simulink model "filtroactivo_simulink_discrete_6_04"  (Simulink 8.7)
settings: Solver=ode45  StartTime=0.0  StopTime=stopTime  RelTol=1e-3
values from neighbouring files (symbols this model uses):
  C_LPF = 90e-6;5e-6;1e-6    [filtroactivo_simulink_discrete_6_default_values.m]    (also in filtroactivo_simulink_opt16_default_values.m; filtroactivo_LPF_C.m = 5.7e-06; filtroactivo_LPF_C_1.m = C; filtroactivo_LPF_C_2.m = 1.67e-05)
  close_net_switch_time = 1    [filtroactivo_simulink_discrete_6_default_values.m]
  control_current_start_time = close_net_switch_time    (= 1)    [filtroactivo_simulink_discrete_6_default_values.m]
  Iload_dephase = 0*pi/180 * [1 0 0 0 0 0 0]    [filtroactivo_simulink_discrete_6_default_values.m]    (also in filtroactivo_simulink_opt16_default_values.m)
  Iload_freq = 50*[1 5 7 11 13 17 19]    [filtroactivo_simulink_discrete_6_default_values.m]    (also in filtroactivo_simulink_opt16_default_values.m)
  Iload_peak = 16*sqrt(2)/100*[100 10 10 10 10 0 0]    [filtroactivo_simulink_discrete_6_default_values.m]    (also in filtroactivo_simulink_opt16_default_values.m)
  Iload_sampletime = 1e-6    (= 1e-06)    [filtroactivo_simulink_discrete_6_default_values.m]    (also in filtroactivo_simulink_opt16_default_values.m)
  Iload_simetric = [-1 1 -1 1 -1 1 -1]    [filtroactivo_simulink_discrete_6_default_values.m]    (also in filtroactivo_simulink_opt16_default_values.m)
  k_I_dqPLL = 0.05/pi    (= 0.0159154943092)    [filtroactivo_simulink_discrete_6_default_values.m]
  k_I_DVcc = 1e-3;1e-1    [filtroactivo_simulink_discrete_6_default_values.m]
  k_P_dqPLL = 0.05/pi    (= 0.0159154943092)    [filtroactivo_simulink_discrete_6_default_values.m]
  k_P_DVcc = 1e-4;2.5e-4;1e-2    [filtroactivo_simulink_discrete_6_default_values.m]
  L_grid = 15e-6    (= 1.5e-05)    [filtroactivo_simulink_discrete_6_default_values.m]    (also in filtroactivo_simulink_opt16_default_values.m; filtroactivo_LPF_C_2.m)
  L_LPF = L    (= 0.004)    [filtroactivo_LPF_C.m]    (also in filtroactivo_LPF_C_1.m = L; filtroactivo_LPF_L.m = 0.001)
  loopPeriod = period_control_current    [filtroactivo_simulink_discrete_6_default_values.m]
  period_control_plant = 0.5e-6    (= 5e-07)    [filtroactivo_simulink_discrete_6_default_values.m]
  period_control_switch = 2e-6    (= 2e-06)    [filtroactivo_simulink_discrete_6_default_values.m]
  R_C_LPF = .1;.5    [filtroactivo_simulink_discrete_6_default_values.m]    (also in filtroactivo_simulink_opt16_default_values.m; filtroactivo_LPF_C.m = 0.5; filtroactivo_LPF_C_2.m = 0.5)
  R_grid = 20e-3    (= 0.02)    [filtroactivo_simulink_discrete_6_default_values.m]    (also in filtroactivo_simulink_opt16_default_values.m; filtroactivo_LPF_C_2.m)
  R_L_LPF = .65;.125    [filtroactivo_simulink_discrete_6_default_values.m]    (also in filtroactivo_simulink_opt16_default_values.m; filtroactivo_LPF_C.m = 0.5)
  R_neutro_inverter_C_LPF = 1e-2;1;50;1e-2    [filtroactivo_simulink_discrete_6_default_values.m]    (also in filtroactivo_simulink_opt16_default_values.m)
  Vcc_desired = 900    [filtroactivo_simulink_discrete_6_default_values.m]    (also in filtroactivo_simulink_opt16_default_values.m)
  Vnet_dephase = 0*pi/180    (= 0)    [filtroactivo_simulink_discrete_6_default_values.m]    (also in filtroactivo_simulink_opt16_default_values.m)
  Vnet_freq = 50    [filtroactivo_simulink_discrete_6_default_values.m]    (also in filtroactivo_simulink_opt16_default_values.m)
  Vnet_peak = 566    [filtroactivo_simulink_discrete_6_default_values.m]    (also in filtroactivo_simulink_opt16_default_values.m)
undefined symbols (not defined in the file or in its folder): period_control_current
libraries: powerlib x50

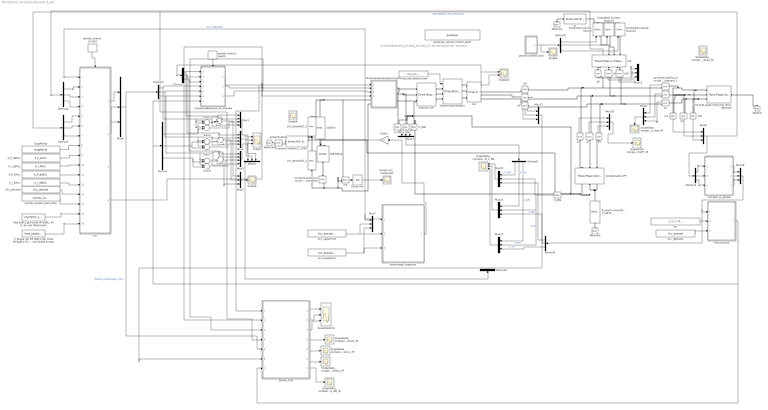
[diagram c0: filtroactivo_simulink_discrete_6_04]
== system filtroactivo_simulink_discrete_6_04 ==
  note: tic,sim('filtroactivo_simulink_discrete_2');,toc load gong.mat; sound(y);
  50Ohm : powerlib/Elements/Series RLC Branch  LConnTagsString=__new0  RConnTagsString=__new0  BranchType=R  Resistance=50  Inductance=1e-3  SetiL0=off  InitialCurrent=0  Capacitance=1e-6  Setx0=off  InitialVoltage=0  Measurements=None
  Condensator LPF : powerlib/Elements/Three-Phase Series RLC Branch  LConnTagsString=A|B|C  RConnTagsString=A|B|C  BranchType=RC  Resistance=R_C_LPF  Inductance=1e-3  Capacitance=C_LPF  Measurements=None
  Controlled Current Source : powerlib/Electrical Sources/Controlled Current Source  Initialize=off  Source_Type=AC  Amplitude=0  Phase=0  Frequency=0  Measurements=None
  Controlled Current Source1 : powerlib/Electrical Sources/Controlled Current Source  Initialize=off  Source_Type=AC  Amplitude=0  Phase=0  Frequency=0  Measurements=None
  Controlled Current Source2 : powerlib/Electrical Sources/Controlled Current Source  Initialize=off  Source_Type=AC  Amplitude=0  Phase=0  Frequency=0  Measurements=None
  Delay Vdc : UnitDelay  InitialCondition=Vcc_desired  SampleTime=-1
  Demux{,1..9} (10 alike) : Demux  Outputs=3
  Gain1 : Gain
  Grid Vnet_peak Vnet_freq Vnet_dephase : powerlib/Electrical Sources/Three-Phase Source  InternalConnection=Yn  VoltagePhases=off  Voltage=Vnet_peak/sqrt(2)  PhaseAngle=Vnet_dephase/pi*180  Voltage_phases=[25e3 25e3 25e3]/sqrt(3)  PhaseAngles_phases=[0 -120 +120]  Frequency=Vnet_freq  NonIdealSource=on  SpecifyImpedance=off  Resistance=R_grid  Inductance=L_grid  ShortCircuitLevel=100e6  BaseVoltage=25e3  XRratio=7  BusType=swing  Pref=0  Qref=0  Prefabc=[10e3, 10e3, 10e3]  Qrefabc=[0, 0, 0]  Qmin=-inf  Qmax=inf
  HB_calculus : MATLAB Function  TreatAsAtomicUnit=on
  IGBT/Diode : powerlib/Power Electronics/IGBT//Diode  Ron=1e-3  Rs=1e5  Cs=inf  Measurements=off
  Inductor LPF : powerlib/Elements/Three-Phase Series RLC Branch  LConnTagsString=A|B|C  RConnTagsString=A|B|C  BranchType=RL  Resistance=R_L_LPF  Inductance=L_LPF  Capacitance=1e-6  Measurements=None
  MOVIE_FCN : MATLAB Function  TreatAsAtomicUnit=on
  Mux1 : Mux
  Mux{5..18} (14 alike) : Mux  Inputs=3
  Mux2 : Mux
  Mux3 : Mux
  Neutral : powerlib/Elements/Neutral  LConnTagsString=a  NodeNumber=1
  Neutral1 : powerlib/Elements/Neutral  LConnTagsString=a  NodeNumber=2
  Neutral2 : powerlib/Elements/Neutral  LConnTagsString=a  NodeNumber=2
  Neutral4 : powerlib/Elements/Neutral  LConnTagsString=a  NodeNumber=2
  R : powerlib/Elements/Series RLC Branch  LConnTagsString=__new0  RConnTagsString=__new0  BranchType=R  Resistance=1  Inductance=1e-3  SetiL0=off  InitialCurrent=0  Capacitance=1e-6  Setx0=off  InitialVoltage=0  Measurements=None
  R_neutro_inverter_C_LPF/2 : powerlib/Elements/Series RLC Branch  LConnTagsString=__new0  RConnTagsString=__new0  BranchType=R  Resistance=R_neutro_inverter_C_LPF/2  Inductance=1e-3  SetiL0=off  InitialCurrent=0  Capacitance=1e-6  Setx0=off  InitialVoltage=0  Measurements=None
  R_neutro_inverter_C_LPF/2 _ : powerlib/Elements/Series RLC Branch  LConnTagsString=__new0  RConnTagsString=__new0  BranchType=R  Resistance=R_neutro_inverter_C_LPF/2  Inductance=1e-3  SetiL0=off  InitialCurrent=0  Capacitance=1e-6  Setx0=off  InitialVoltage=0  Measurements=None
  Scope1 : Scope
  Scope10 : Scope  NumInputPorts=2
  Scope4 : Scope
  Scope6 : Scope
  Scope7 : Scope  NumInputPorts=3
  ScopeData_compensator_Subsystem__Scope_HB_3F : Scope
  ScopeData_compensator_Subsystem__Scope_ICLPF_3F : Scope
  ScopeData_compensator_Subsystem__Scope_Iinversor_3F : Scope
  ScopeData_compensator_Subsystem__Scope_Iinversorreference_3F : Scope
  ScopeData_compensator_Subsystem__Scope_Iload_3F : Scope
  ScopeData_compensator_Subsystem__Scope_Inet_3F : Scope
  ScopeData_compensator_Subsystem__Scope_V_UN_V_MN_V_RN : Scope  NumInputPorts=3
  ScopeData_compensator_Subsystem__Scope_Vnet_measured_3F : Scope
  ScopeSwitchs : Scope  NumInputPorts=3
  Scope_Vcc_measured : Scope
  Sum1 : Sum  Inputs=+-
  Sum2 : Sum  Inputs=-+|
  Sum3 : Sum
  Sum4 : Sum  Inputs=-+|
  Sum5 : Sum  Inputs=-+|
  Sum6 : Sum  Inputs=+-
  Sum7 : Sum
  Sum8 : Sum  Inputs=+-
  Sum9 : Sum
  Three-Phase Breaker : powerlib/Elements/Three-Phase Breaker  InitialState=open  SwitchA=on  SwitchB=on  SwitchC=on  SwitchTimes=[0.020]  External=on  BreakerResistance=0.001  SnubberResistance=1e6  SnubberCapacitance=inf  Measurements=None
  Three-phase two-level inverter : Subsystem
  V_MN : powerlib/Measurements/Voltage Measurement  PhasorSimulation=off  OutputType=Complex  PSBequivalent=0
  V_UN : powerlib/Measurements/Voltage Measurement  PhasorSimulation=off  OutputType=Complex  PSBequivalent=0
  V_VN : powerlib/Measurements/Voltage Measurement  PhasorSimulation=off  OutputType=Complex  PSBequivalent=0
  V_WN : powerlib/Measurements/Voltage Measurement  PhasorSimulation=off  OutputType=Complex  PSBequivalent=0
  "V_phase-net Vd dqPLL got noise till dqPLL fix it, we use Vpeak known" : Constant  Value=Vnet_peak/sqrt(3)
  Vcc_desired : Constant  Value=Vcc_desired
  Vcc_desired/2_1 : powerlib/Elements/Series RLC Branch  LConnTagsString=__new0  RConnTagsString=__new0  BranchType=C  Resistance=0  Inductance=0  SetiL0=off  InitialCurrent=0  Capacitance=1e-2  Setx0=on  InitialVoltage=Vcc_desired/2  Measurements=None
  Vcc_desired/2_2 : powerlib/Elements/Series RLC Branch  LConnTagsString=__new0  RConnTagsString=__new0  BranchType=C  Resistance=0  Inductance=0  SetiL0=off  InitialCurrent=0  Capacitance=1e-2  Setx0=on  InitialVoltage=Vcc_desired/2  Measurements=None
  Vcc_desired1 : Constant  Value=Vcc_desired
  Vcc_lowerlimit : Constant  Value=Vcc_desired * 101 / 100
  Vcc_upperlimit : Constant  Value=Vcc_desired * 105 / 100
  a{,1..10} (11 alike) : powerlib/Measurements/Current Measurement  PhasorSimulation=off  OutputType=Complex  PSBequivalent=0
  amperimeter4 : powerlib/Measurements/Current Measurement  PhasorSimulation=off  OutputType=Complex  PSBequivalent=0
  close_net_switch_time : Constant  Value=close_net_switch_time
  complex_to_phase : MATLAB Function  TreatAsAtomicUnit=on
  control_current_start_time : Constant  Value=control_current_start_time
  "corriente positiva si va del + al - del block Current Measurement " : powerlib/Measurements/Current Measurement  PhasorSimulation=off  OutputType=Complex  PSBequivalent=0
  corriente positiva si va del + al - del block Current Measurement 1 : powerlib/Measurements/Current Measurement  PhasorSimulation=off  OutputType=Complex  PSBequivalent=0
  fcn : Subsystem
  "freq dqPLL got noise till dqPLL fix it, we use freq known" : Constant  Value=2*pi*50*C_LPF
  kH : Constant  Value=1 / ( 2 * 0.005 * 25e3 *Vcc_desired )
  k_I_DVcc : Constant  Value=k_I_dqPLL
  k_I_dqPLL : Constant  Value=k_I_DVcc
  k_P_DVcc : Constant  Value=k_P_dqPLL
  k_P_dqPLL : Constant  Value=k_P_DVcc
  loopPeriod : Constant  Value=loopPeriod
  m{1,3,5,8} (4 alike) : powerlib/Measurements/Voltage Measurement  PhasorSimulation=off  OutputType=Complex  PSBequivalent=0
  m2 : powerlib/Measurements/Three-Phase V-I Measurement  VoltageMeasurement=phase-to-phase  SetLabelV=off  LabelV=Vabc  Vpu=off  VpuLL=off  CurrentMeasurement=yes  SetLabelI=off  LabelI=Iabc  Ipu=off  Pbase=100e6  Vbase=500e3  OutputType=Complex  PhasorSimulation=off  PSBequivalent=0
  m6 : powerlib/Measurements/Three-Phase V-I Measurement  VoltageMeasurement=phase-to-phase  SetLabelV=off  LabelV=Vabc  Vpu=off  VpuLL=off  CurrentMeasurement=yes  SetLabelI=off  LabelI=Iabc  Ipu=off  Pbase=100e6  Vbase=500e3  OutputType=Complex  PhasorSimulation=off  PSBequivalent=0
  measured&desired_to_SuSvSw : Subsystem
  overcharge_capacitor : MATLAB Function  TreatAsAtomicUnit=on
  period_control_current : DiscretePulseGenerator  PulseType=Time based  Period=period_control_current  PulseWidth=50
  period_control_switch : DiscretePulseGenerator  PulseType=Time based  Period=period_control_switch  PulseWidth=50
  phase currents load : Subsystem
  powergui_period_control_plant : powerlib/powergui  Priority=1  SimulationMode=Discrete  SolverType=Tustin  SampleTime=period_control_plant  frequency=60  SPID=off  DisableSnubberDevices=off  DisableRonSwitches=off  DisableVfSwitches=off  SwTol=0  DisplayEquations=off  Interpol=off  ExternalGateDelay=off  methode=off  Ts=10  FunctionMessages=off  echomessages=off  HookPort=off  EnableUseOfTLC=off  x0status=blocks  frequencyindice=0  Pbase=100e6  ErrMax=1e-4  Iterations=50  UnitsV=kV  UnitsW=MW  buscounter=0  RestoreLinks=warning  ResistiveCurrentMeasurement=off  Frange=[0:2:500]  Ylog=off  Xlog=on  ShowGrid=off  save=off  variable=ZData  structure=ScopeData_compensator_Subsystem__Scope11  ZoomFFT=off  StartTime=4.72  cycles=14  DisplayStyle=3  fundamental=50  FreqAxis=on  MaxFrequency=40*50  frequencyindicesteady=1  RmsSteady=1  display=off
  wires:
  period_control_switch/1 -> measured&desired_to_SuSvSw/Trigger
  Demux2/1 -> measured&desired_to_SuSvSw/4(Iu*), Sum2/2, Mux1/2, Sum1/1, Sum3/1
  Demux2/2 -> measured&desired_to_SuSvSw/5(Iv*), Sum7/1, Sum6/1, Mux2/2, Sum4/2
  Demux2/3 -> measured&desired_to_SuSvSw/6(Iw*), Sum9/1, Sum8/1, Mux3/2, Sum5/2
  Mux1/1 -> Mux16/1, Scope7/1
  Sum1/1 -> Mux1/4
  Sum3/1 -> Mux1/3
  Mux2/1 -> Scope7/2, Mux16/2
  Mux3/1 -> Mux16/3, Scope7/3
  Sum6/1 -> Mux2/3
  Sum8/1 -> Mux3/3
  Demux/1 -> Sum1/2, Sum3/2
  Demux/2 -> Sum6/2, Sum7/2
  Demux/3 -> Sum9/2, Sum8/2
  m3/1 -> Delay Vdc/1
  HB_calculus/1(HB) -> MOVIE_FCN/7(g), Demux/1, measured&desired_to_SuSvSw/7(H)
  m2/1 -> Scope10/2
  Mux9/1 -> MOVIE_FCN/4(d), Demux7/1, Demux3/1  "Vphasephase_net_measured"
  Demux1/2 -> Sum4/1, Mux2/1, measured&desired_to_SuSvSw/2(Iv)
  Demux1/3 -> measured&desired_to_SuSvSw/3(Iw), Sum5/1, Mux3/1
  Demux1/1 -> Sum2/1, Mux1/1, measured&desired_to_SuSvSw/1(Iu)
  Demux5/1 -> Controlled Current Source/1
  Demux5/2 -> Controlled Current Source1/1
  Demux5/3 -> Controlled Current Source2/1
  phase currents load/1(Out1) -> Scope1/1, Demux5/1
  Mux5/1 -> Scope6/1
  Sum2/1 -> Mux5/1
  Sum4/1 -> Mux5/2
  Sum5/1 -> Mux5/3
  Sum7/1 -> Mux2/4
  Sum9/1 -> Mux3/4
  m2/2 -> Scope10/1, Demux1/1
  Mux6/1 -> MOVIE_FCN/5(e), Demux2/1  "Iphase_compensator_reference"
  amperimeter4/1 -> ?
  Delay Vdc/1 -> fcn/1(Vcc_measured), Scope_Vcc_measured/1, overcharge_capacitor/1(Vcc_measured), Mux7/1  "Vcc_measured"
  period_control_current/1 -> fcn/Trigger
  fcn/2(Iv_ref) -> Mux6/2
  fcn/3(Iw_ref) -> Mux6/3
  fcn/1(Iu_ref) -> Mux6/1
  m6/2 -> Demux4/1
  Demux4/1 -> fcn/2(Ia_load)
  close_net_switch_time/1 -> Three-Phase Breaker/1
  fcn/4(activate_poles) -> Three-phase two-level inverter/4(activate_poles)
  Vcc_upperlimit/1 -> overcharge_capacitor/2(Vcc_upperlimit), Mux7/2
  Vcc_lowerlimit/1 -> overcharge_capacitor/3(Vcc_lowerlimit), Mux7/3
  overcharge_capacitor/1(pSfrenado) -> Gain1/1
  Gain1/1 -> IGBT/Diode/1
  Mux7/1 -> ?
  "corriente positiva si va del + al - del block Current Measurement "/1 -> ?
  Mux8/1 -> ScopeData_compensator_Subsystem__Scope_Inet_3F/1
  corriente positiva si va del + al - del block Current Measurement 1/1 -> Mux8/1
  a/1 -> Mux8/2
  a1/1 -> Mux8/3
  m1/1 -> Mux9/1
  m5/1 -> Mux9/2
  m8/1 -> Mux9/3
  Mux10/1 -> ScopeData_compensator_Subsystem__Scope_ICLPF_3F/1
  a2/1 -> Mux10/1
  a3/1 -> Mux10/2
  a4/1 -> Mux10/3
  Mux11/1 -> MOVIE_FCN/6(f)
  a5/1 -> Mux11/1
  a6/1 -> Mux11/2
  a7/1 -> Mux11/3
  Mux12/1 -> ?
  a10/1 -> Mux12/3
  a9/1 -> Mux12/2
  a8/1 -> Mux12/1
  control_current_start_time/1 -> fcn/14(control_current_start_time)
  loopPeriod/1 -> fcn/8(loopPeriod)
  k_P_DVcc/1 -> fcn/11(k_P_dqPLL)
  k_I_DVcc/1 -> fcn/12(k_I_dqPLL)
  k_I_dqPLL/1 -> fcn/10(k_I_DVcc)
  k_P_dqPLL/1 -> fcn/9(k_P_DVcc)
  "freq dqPLL got noise till dqPLL fix it, we use freq known"/1 -> fcn/15(X_C_LPF)
  "V_phase-net Vd dqPLL got noise till dqPLL fix it, we use Vpeak known"/1 -> fcn/16(Vpeak_arbitrary)
  Vcc_desired/1 -> fcn/13(Vcc_desired)
  Demux4/2 -> fcn/3(Ib_load)
  Demux4/3 -> fcn/4(Ic_load)
  Demux7/1 -> fcn/5(Va)
  Demux7/2 -> fcn/6(Vb)
  Demux7/3 -> fcn/7(Vc)
  Mux13/1 -> ScopeData_compensator_Subsystem__Scope_V_UN_V_MN_V_RN/1
  Demux3/2 -> complex_to_phase/2(Vst)
  Demux3/1 -> complex_to_phase/1(Vrs)
  Demux3/3 -> complex_to_phase/3(Vtr)
  measured&desired_to_SuSvSw/3(Sw) -> MOVIE_FCN/3(c), Three-phase two-level inverter/3(Sc)
  measured&desired_to_SuSvSw/2(Sv) -> MOVIE_FCN/2(b), Three-phase two-level inverter/2(Sb)
  measured&desired_to_SuSvSw/1(Su) -> MOVIE_FCN/1(a), Three-phase two-level inverter/1(Sa)
  Mux14/1 -> ScopeData_compensator_Subsystem__Scope_V_UN_V_MN_V_RN/2
  Mux16/1 -> Demux6/1
  V_VN/1 -> Mux17/2
  V_WN/1 -> Mux17/3
  V_UN/1 -> Mux17/1
  V_MN/1 -> Mux15/2, Mux14/2, Mux13/2  "V_MN"
  Mux17/1 -> Demux8/1
  Demux8/1 -> Mux13/1  "V_UN"
  Demux8/2 -> Mux14/1  "V_VN"
  Demux8/3 -> Mux15/1  "V_WN"
  complex_to_phase/2(Vs) -> Mux18/2
  complex_to_phase/1(Vr) -> Mux18/1
  complex_to_phase/3(Vt) -> Mux18/3
  Mux18/1 -> Demux9/1, HB_calculus/1(Vfaseneutro)
  Demux9/1 -> Mux13/3  "V_RN"
  Demux9/2 -> Mux14/3  "V_SN"
  Demux9/3 -> Mux15/3  "V_TN"
  Demux6/1 -> ?  "I_U"
  Demux6/2 -> ?  "I_V"
  Demux6/3 -> ?  "I_W"
  Mux15/1 -> ScopeData_compensator_Subsystem__Scope_V_UN_V_MN_V_RN/3
  kH/1 -> HB_calculus/2(Kh)
  Vcc_desired1/1 -> HB_calculus/3(Vcc_desired)
  MOVIE_FCN/1(a1) -> ScopeSwitchs/1
  MOVIE_FCN/2(b1) -> ScopeSwitchs/2
  MOVIE_FCN/3(c1) -> ScopeSwitchs/3
  MOVIE_FCN/4(d1) -> ScopeData_compensator_Subsystem__Scope_Vnet_measured_3F/1
  MOVIE_FCN/5(e1) -> ScopeData_compensator_Subsystem__Scope_Iinversorreference_3F/1
  MOVIE_FCN/6(f1) -> ScopeData_compensator_Subsystem__Scope_Iinversor_3F/1
  MOVIE_FCN/7(g1) -> ScopeData_compensator_Subsystem__Scope_HB_3F/1
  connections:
  Vcc_desired/2_2/RConn1 -- "corriente positiva si va del + al - del block Current Measurement "/RConn1 -- Three-phase two-level inverter/LConn2 -- m3/LConn2
  Three-phase two-level inverter/LConn1 -- 50Ohm/RConn1 -- Vcc_desired/2_1/LConn1 -- m3/LConn1
  corriente positiva si va del + al - del block Current Measurement 1/RConn1 -- a8/RConn1 -- a2/RConn1 -- a5/RConn1
  Controlled Current Source/RConn1 -- Controlled Current Source1/RConn1 -- Controlled Current Source2/RConn1 -- R/RConn1
  a/RConn1 -- a9/RConn1 -- a3/RConn1 -- a6/RConn1
  a1/RConn1 -- a4/RConn1 -- a7/RConn1 -- a10/RConn1
  Condensator LPF/RConn2 -- V_WN/LConn2 -- V_VN/LConn2 -- V_UN/LConn2 -- V_MN/LConn2 -- Condensator LPF/RConn1 -- Condensator LPF/RConn3 -- R_neutro_inverter_C_LPF/2 _/RConn1
  Vcc_desired/2_1/RConn1 -- Vcc_desired/2_2/LConn1 -- V_MN/LConn1 -- R_neutro_inverter_C_LPF/2/RConn1
  Three-phase two-level inverter/RConn1 -- V_UN/LConn1 -- Inductor LPF/LConn1
  Three-phase two-level inverter/RConn2 -- V_VN/LConn1 -- Inductor LPF/LConn2
  m6/RConn1 -- Controlled Current Source/LConn1
  Neutral1/LConn1 -- R/LConn1
  Grid Vnet_peak Vnet_freq Vnet_dephase/RConn2 -- m1/LConn2 -- a/LConn1 -- m5/LConn1
  Grid Vnet_peak Vnet_freq Vnet_dephase/LConn1 -- Neutral/LConn1
  Inductor LPF/RConn3 -- Three-Phase Breaker/LConn3
  Inductor LPF/RConn1 -- Three-Phase Breaker/LConn1
  Grid Vnet_peak Vnet_freq Vnet_dephase/RConn1 -- m8/LConn2 -- m1/LConn1 -- corriente positiva si va del + al - del block Current Measurement 1/LConn1
  m2/LConn1 -- Three-Phase Breaker/RConn1
  m6/RConn2 -- Controlled Current Source1/LConn1
  Inductor LPF/RConn2 -- Three-Phase Breaker/LConn2
  m2/LConn3 -- Three-Phase Breaker/RConn3
  m2/LConn2 -- Three-Phase Breaker/RConn2
  m6/RConn3 -- Controlled Current Source2/LConn1
  R_neutro_inverter_C_LPF/2 _/LConn1 -- Neutral2/LConn1
  Inductor LPF/LConn3 -- V_WN/LConn1 -- Three-phase two-level inverter/RConn3
  Grid Vnet_peak Vnet_freq Vnet_dephase/RConn3 -- m8/LConn1 -- m5/LConn2 -- a1/LConn1
  amperimeter4/LConn1 -- Neutral4/LConn1
  R_neutro_inverter_C_LPF/2/LConn1 -- amperimeter4/RConn1
  50Ohm/LConn1 -- IGBT/Diode/LConn1
  "corriente positiva si va del + al - del block Current Measurement "/LConn1 -- IGBT/Diode/RConn1
  a3/LConn1 -- Condensator LPF/LConn2
  Condensator LPF/LConn3 -- a4/LConn1
  a2/LConn1 -- Condensator LPF/LConn1
  a6/LConn1 -- m2/RConn2
  a5/LConn1 -- m2/RConn1
  a7/LConn1 -- m2/RConn3
  a8/LConn1 -- m6/LConn1
  a9/LConn1 -- m6/LConn2
  a10/LConn1 -- m6/LConn3

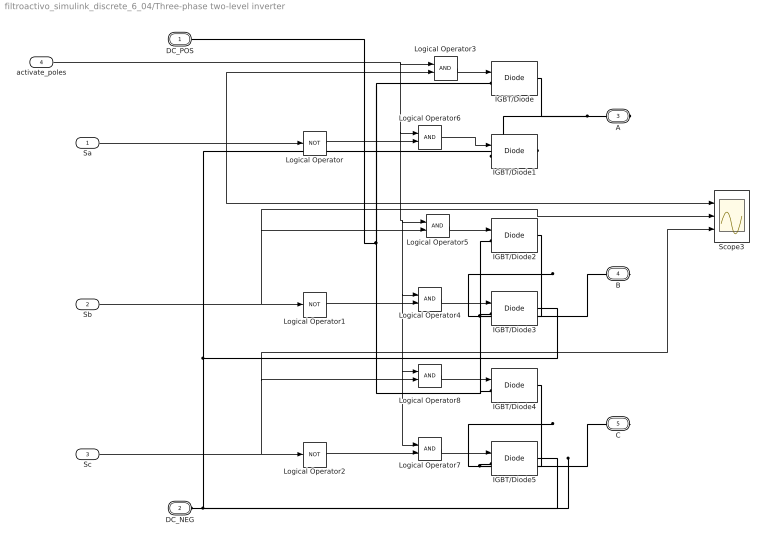
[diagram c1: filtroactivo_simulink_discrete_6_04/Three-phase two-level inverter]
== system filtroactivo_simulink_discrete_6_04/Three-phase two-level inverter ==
  Sa : Inport
  Sb : Inport  Port=2
  Sc : Inport  Port=3
  activate_poles : Inport  Port=4
  IGBT/Diode{,1..5} (6 alike) : powerlib/Power Electronics/IGBT//Diode  Ron=1e-3  Rs=1e5  Cs=inf  Measurements=off
  Logical Operator : Logic  Operator=NOT  AllPortsSameDT=off  OutDataTypeStr=boolean
  Logical Operator1 : Logic  Operator=NOT  AllPortsSameDT=off  OutDataTypeStr=boolean
  Logical Operator2 : Logic  Operator=NOT  AllPortsSameDT=off  OutDataTypeStr=boolean
  Logical Operator{3..8} (6 alike) : Logic  AllPortsSameDT=off  OutDataTypeStr=boolean
  Scope3 : Scope  NumInputPorts=3
  DC_POS : PMIOPort  Tag=PMCPort  Port=1  Side=Left
  DC_NEG : PMIOPort  Tag=PMCPort  Port=2  Side=Left
  A : PMIOPort  Tag=PMCPort  Port=3  Side=Right
  B : PMIOPort  Tag=PMCPort  Port=4  Side=Right
  C : PMIOPort  Tag=PMCPort  Port=5  Side=Right
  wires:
  Sc/1 -> Scope3/3, Logical Operator8/2, Logical Operator2/1
  Logical Operator2/1 -> Logical Operator7/2
  Sb/1 -> Scope3/2, Logical Operator5/2, Logical Operator1/1
  Sa/1 -> Scope3/1, Logical Operator3/2, Logical Operator/1
  activate_poles/1 -> Logical Operator6/1, Logical Operator7/1, Logical Operator8/1, Logical Operator4/1, Logical Operator5/1, Logical Operator3/1
  Logical Operator3/1 -> IGBT/Diode/1
  Logical Operator/1 -> Logical Operator6/2
  Logical Operator6/1 -> IGBT/Diode1/1
  Logical Operator1/1 -> Logical Operator4/2
  Logical Operator4/1 -> IGBT/Diode3/1
  Logical Operator5/1 -> IGBT/Diode2/1
  Logical Operator7/1 -> IGBT/Diode5/1
  Logical Operator8/1 -> IGBT/Diode4/1
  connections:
  IGBT/Diode5/LConn1 -- IGBT/Diode4/RConn1 -- C/RConn1
  IGBT/Diode3/LConn1 -- B/RConn1 -- IGBT/Diode2/RConn1
  IGBT/Diode4/LConn1 -- IGBT/Diode2/LConn1 -- DC_POS/RConn1 -- IGBT/Diode/LConn1
  A/RConn1 -- IGBT/Diode1/LConn1 -- IGBT/Diode/RConn1
  DC_NEG/RConn1 -- IGBT/Diode5/RConn1 -- IGBT/Diode3/RConn1 -- IGBT/Diode1/RConn1

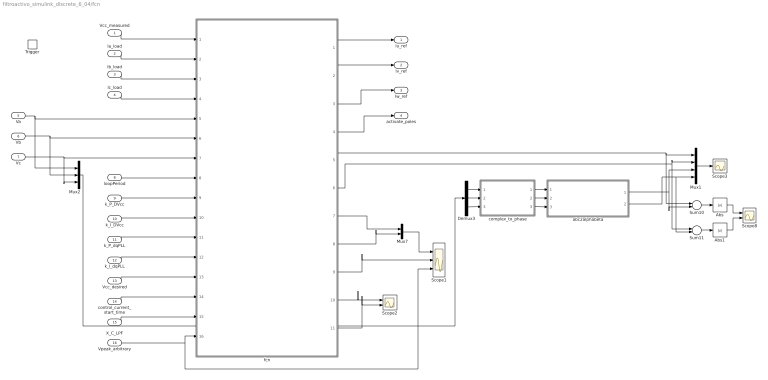
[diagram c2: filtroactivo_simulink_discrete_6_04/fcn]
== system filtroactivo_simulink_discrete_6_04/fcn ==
  Vcc_measured : Inport
  Ia_load : Inport  Port=2
  Ib_load : Inport  Port=3
  Ic_load : Inport  Port=4
  Va : Inport  Port=5
  Vb : Inport  Port=6
  Vc : Inport  Port=7
  loopPeriod : Inport  Port=8
  k_P_DVcc : Inport  Port=9
  k_I_DVcc : Inport  Port=10
  k_P_dqPLL : Inport  Port=11
  k_I_dqPLL : Inport  Port=12
  Vcc_desired : Inport  Port=13
  control_current_start_time : Inport  Port=14
  X_C_LPF : Inport  Port=15
  Vpeak_arbitrary : Inport  Port=16
  Trigger : TriggerPort  VariantControl=Variant
  Abs : Abs
  Abs1 : Abs
  Demux3 : Demux  Outputs=3
  Mux1 : Mux
  Mux2 : Mux  Inputs=3
  Mux7 : Mux  Inputs=2
  Scope1 : Scope  NumInputPorts=3
  Scope2 : Scope  NumInputPorts=2
  Scope3 : Scope
  Scope8 : Scope  NumInputPorts=2
  Sum10 : Sum  Inputs=+-
  Sum11 : Sum  Inputs=+-
  abc2alphabeta : MATLAB Function  TreatAsAtomicUnit=on
  complex_to_phase : MATLAB Function  TreatAsAtomicUnit=on
  fcn : MATLAB Function  TreatAsAtomicUnit=on
  Iu_ref : Outport
  Iv_ref : Outport  Port=2
  Iw_ref : Outport  Port=3
  activate_poles : Outport  Port=4
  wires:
  Vc/1 -> Mux2/3, fcn/7(Vc)
  Vb/1 -> Mux2/2, fcn/6(Vb)
  Ic_load/1 -> fcn/4(Ic_load)
  Va/1 -> Mux2/1, fcn/5(Va)
  Ib_load/1 -> fcn/3(Ib_load)
  Ia_load/1 -> fcn/2(Ia_load)
  Vcc_measured/1 -> fcn/1(Vcc_measured)
  loopPeriod/1 -> fcn/8(loopPeriod)
  k_P_DVcc/1 -> fcn/9(k_P_DVcc)
  k_I_DVcc/1 -> fcn/10(k_I_DVcc)
  Vpeak_arbitrary/1 -> fcn/16(Vpeak_arbitrary), Scope1/3
  fcn/2(Iv_ref) -> Iv_ref/1
  fcn/3(Iw_ref) -> Iw_ref/1
  fcn/4(activate_poles) -> activate_poles/1
  fcn/1(Iu_ref) -> Iu_ref/1
  Mux7/1 -> Scope1/1
  fcn/7(control_current_start_counter_output) -> Mux7/1
  fcn/8(control_current_start_counter_max_output) -> Mux7/2
  fcn/9(DVcc) -> Scope1/2
  fcn/10(DVcc_afterPI) -> Scope2/1
  fcn/11(PI_I_output) -> Scope2/2
  Demux3/1 -> complex_to_phase/1(Vrs)
  Demux3/2 -> complex_to_phase/2(Vst)
  Demux3/3 -> complex_to_phase/3(Vtr)
  complex_to_phase/1(Vr) -> abc2alphabeta/1(a)
  complex_to_phase/2(Vs) -> abc2alphabeta/2(b)
  complex_to_phase/3(Vt) -> abc2alphabeta/3(c)
  Mux1/1 -> Scope3/1
  fcn/6(V_beta) -> Mux1/2, Sum11/1
  fcn/5(V_alpha) -> Sum10/1, Mux1/1
  abc2alphabeta/1(alpha) -> Mux1/3, Sum10/2
  abc2alphabeta/2(beta) -> Sum11/2, Mux1/4
  Sum10/1 -> Abs/1
  Sum11/1 -> Abs1/1
  Abs1/1 -> Scope8/2
  Abs/1 -> Scope8/1
  Mux2/1 -> Demux3/1
  k_I_dqPLL/1 -> fcn/12(k_I_dqPLL)
  k_P_dqPLL/1 -> fcn/11(k_P_dqPLL)
  X_C_LPF/1 -> fcn/15(X_C_LPF)
  Vcc_desired/1 -> fcn/13(Vcc_desired)
  control_current_start_time/1 -> fcn/14(control_current_start_time)

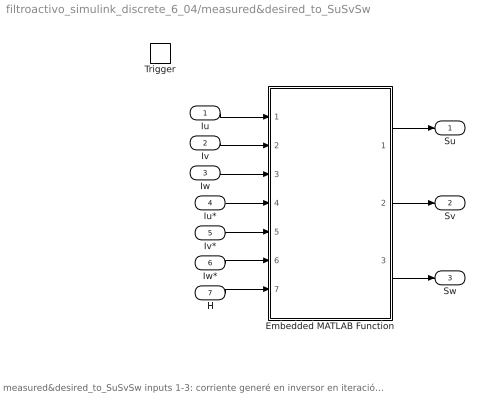
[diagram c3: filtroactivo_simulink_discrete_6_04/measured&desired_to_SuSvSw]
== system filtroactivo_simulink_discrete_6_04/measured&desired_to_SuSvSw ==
  note: measured&desired_to_SuSvSw inputs 1-3: corriente generé en inversor en iteración anterior inputs 4-6: corriente q deseo generar en inversor outputs: disparos Su,Sv,Sw q definen la corriente mas parecida a deseada que puedo generar
  Iu : Inport
  Iv : Inport  Port=2
  Iw : Inport  Port=3
  Iu* : Inport  Port=4
  Iv* : Inport  Port=5
  Iw* : Inport  Port=6
  H : Inport  Port=7
  Trigger : TriggerPort  VariantControl=Variant
  Embedded MATLAB Function : MATLAB Function  TreatAsAtomicUnit=on
  Su : Outport
  Sv : Outport  Port=2
  Sw : Outport  Port=3
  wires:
  Embedded MATLAB Function/3(Sw) -> Sw/1
  Embedded MATLAB Function/2(Sv) -> Sv/1
  Embedded MATLAB Function/1(Su) -> Su/1
  Iu/1 -> Embedded MATLAB Function/1(Iu)
  Iv/1 -> Embedded MATLAB Function/2(Iv)
  Iw/1 -> Embedded MATLAB Function/3(Iw)
  Iu*/1 -> Embedded MATLAB Function/4(Iu1)
  Iv*/1 -> Embedded MATLAB Function/5(Iv1)
  Iw*/1 -> Embedded MATLAB Function/6(Iw1)
  H/1 -> Embedded MATLAB Function/7(H)

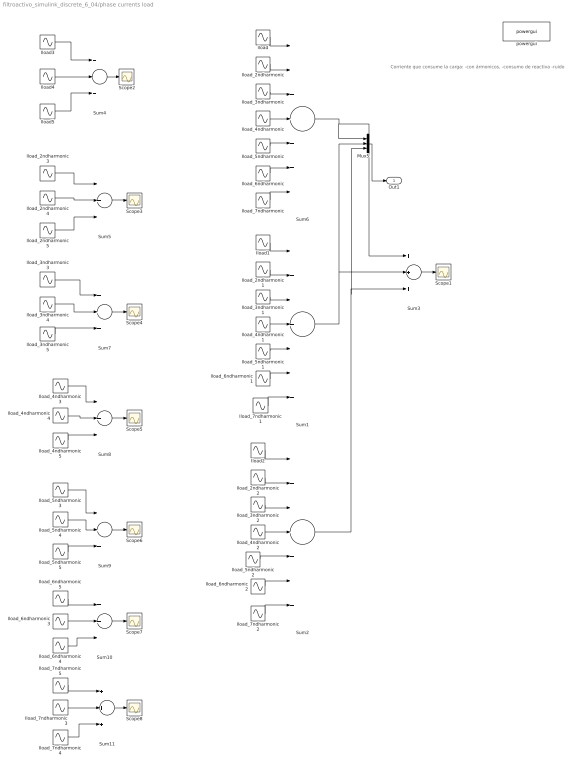
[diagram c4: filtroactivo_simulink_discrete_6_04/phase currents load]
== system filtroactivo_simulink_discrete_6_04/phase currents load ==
  note: Corriente que consume la carga: -con ármonicos, -consumo de reactiva -ruido
  Iload : Sin  Amplitude=Iload_peak(1)  Frequency=2*pi*Iload_freq(1)  Phase=Iload_dephase(1)  SampleTime=Iload_sampletime
  Iload1 : Sin  Amplitude=Iload_peak(1)  Frequency=2*pi*Iload_freq(1)  Phase=Iload_dephase(1) + 2*pi/3*Iload_simetric(1)  SampleTime=Iload_sampletime
  Iload2 : Sin  Amplitude=Iload_peak(1)  Frequency=2*pi*Iload_freq(1)  Phase=Iload_dephase(1) + 4*pi/3*Iload_simetric(1)  SampleTime=Iload_sampletime
  Iload3 : Sin  Amplitude=Iload_peak(1)  Frequency=2*pi*Iload_freq(1)  Phase=Iload_dephase(1)  SampleTime=Iload_sampletime
  Iload4 : Sin  Amplitude=Iload_peak(1)  Frequency=2*pi*Iload_freq(1)  Phase=Iload_dephase(1) + 2*pi/3*Iload_simetric(1)  SampleTime=Iload_sampletime
  Iload5 : Sin  Amplitude=Iload_peak(1)  Frequency=2*pi*Iload_freq(1)  Phase=Iload_dephase(1) + 4*pi/3*Iload_simetric(1)  SampleTime=Iload_sampletime
  Iload_2ndharmonic : Sin  Amplitude=Iload_peak(2)  Frequency=2*pi*Iload_freq(2)  Phase=Iload_dephase(2)  SampleTime=Iload_sampletime
  Iload_2ndharmonic1 : Sin  Amplitude=Iload_peak(2)  Frequency=2*pi*Iload_freq(2)  Phase=Iload_dephase(2) + 2*pi/3*Iload_simetric(2)  SampleTime=Iload_sampletime
  Iload_2ndharmonic2 : Sin  Amplitude=Iload_peak(2)  Frequency=2*pi*Iload_freq(2)  Phase=Iload_dephase(2) + 4*pi/3*Iload_simetric(2)  SampleTime=Iload_sampletime
  Iload_2ndharmonic3 : Sin  Amplitude=Iload_peak(2)  Frequency=2*pi*Iload_freq(2)  Phase=Iload_dephase(2)  SampleTime=Iload_sampletime
  Iload_2ndharmonic4 : Sin  Amplitude=Iload_peak(2)  Frequency=2*pi*Iload_freq(2)  Phase=Iload_dephase(2) + 2*pi/3*Iload_simetric(2)  SampleTime=Iload_sampletime
  Iload_2ndharmonic5 : Sin  Amplitude=Iload_peak(2)  Frequency=2*pi*Iload_freq(2)  Phase=Iload_dephase(2) + 4*pi/3*Iload_simetric(2)  SampleTime=Iload_sampletime
  Iload_3ndharmonic : Sin  Amplitude=Iload_peak(3)  Frequency=2*pi*Iload_freq(3)  Phase=Iload_dephase(3)  SampleTime=Iload_sampletime
  Iload_3ndharmonic1 : Sin  Amplitude=Iload_peak(3)  Frequency=2*pi*Iload_freq(3)  Phase=Iload_dephase(3) + 2*pi/3*Iload_simetric(3)  SampleTime=Iload_sampletime
  Iload_3ndharmonic2 : Sin  Amplitude=Iload_peak(3)  Frequency=2*pi*Iload_freq(3)  Phase=Iload_dephase(3) + 4*pi/3*Iload_simetric(3)  SampleTime=Iload_sampletime
  Iload_3ndharmonic3 : Sin  Amplitude=Iload_peak(3)  Frequency=2*pi*Iload_freq(3)  Phase=Iload_dephase(3)  SampleTime=Iload_sampletime
  Iload_3ndharmonic4 : Sin  Amplitude=Iload_peak(3)  Frequency=2*pi*Iload_freq(3)  Phase=Iload_dephase(3) + 2*pi/3*Iload_simetric(3)  SampleTime=Iload_sampletime
  Iload_3ndharmonic5 : Sin  Amplitude=Iload_peak(3)  Frequency=2*pi*Iload_freq(3)  Phase=Iload_dephase(3) + 4*pi/3*Iload_simetric(3)  SampleTime=Iload_sampletime
  Iload_4ndharmonic : Sin  Amplitude=Iload_peak(4)  Frequency=2*pi*Iload_freq(4)  Phase=Iload_dephase(4)  SampleTime=Iload_sampletime
  Iload_4ndharmonic1 : Sin  Amplitude=Iload_peak(4)  Frequency=2*pi*Iload_freq(4)  Phase=Iload_dephase(4) + 2*pi/3*Iload_simetric(4)  SampleTime=Iload_sampletime
  Iload_4ndharmonic2 : Sin  Amplitude=Iload_peak(4)  Frequency=2*pi*Iload_freq(4)  Phase=Iload_dephase(4) + 4*pi/3*Iload_simetric(4)  SampleTime=Iload_sampletime
  Iload_4ndharmonic3 : Sin  Amplitude=Iload_peak(4)  Frequency=2*pi*Iload_freq(4)  Phase=Iload_dephase(4)  SampleTime=Iload_sampletime
  Iload_4ndharmonic4 : Sin  Amplitude=Iload_peak(4)  Frequency=2*pi*Iload_freq(4)  Phase=Iload_dephase(4) + 2*pi/3*Iload_simetric(4)  SampleTime=Iload_sampletime
  Iload_4ndharmonic5 : Sin  Amplitude=Iload_peak(4)  Frequency=2*pi*Iload_freq(4)  Phase=Iload_dephase(4) + 4*pi/3*Iload_simetric(4)  SampleTime=Iload_sampletime
  Iload_5ndharmonic : Sin  Amplitude=Iload_peak(5)  Frequency=2*pi*Iload_freq(5)  Phase=Iload_dephase(5)  SampleTime=Iload_sampletime
  Iload_5ndharmonic1 : Sin  Amplitude=Iload_peak(5)  Frequency=2*pi*Iload_freq(5)  Phase=Iload_dephase(5) + 2*pi/3*Iload_simetric(5)  SampleTime=Iload_sampletime
  Iload_5ndharmonic2 : Sin  Amplitude=Iload_peak(5)  Frequency=2*pi*Iload_freq(5)  Phase=Iload_dephase(5) + 4*pi/3*Iload_simetric(5)  SampleTime=Iload_sampletime
  Iload_5ndharmonic3 : Sin  Amplitude=Iload_peak(5)  Frequency=2*pi*Iload_freq(5)  Phase=Iload_dephase(5)  SampleTime=Iload_sampletime
  Iload_5ndharmonic4 : Sin  Amplitude=Iload_peak(5)  Frequency=2*pi*Iload_freq(5)  Phase=Iload_dephase(5) + 2*pi/3*Iload_simetric(5)  SampleTime=Iload_sampletime
  Iload_5ndharmonic5 : Sin  Amplitude=Iload_peak(5)  Frequency=2*pi*Iload_freq(5)  Phase=Iload_dephase(5) + 4*pi/3*Iload_simetric(5)  SampleTime=Iload_sampletime
  Iload_6ndharmonic : Sin  Amplitude=Iload_peak(6)  Frequency=2*pi*Iload_freq(6)  Phase=Iload_dephase(6)  SampleTime=Iload_sampletime
  Iload_6ndharmonic1 : Sin  Amplitude=Iload_peak(6)  Frequency=2*pi*Iload_freq(6)  Phase=Iload_dephase(6) + 2*pi/3*Iload_simetric(6)  SampleTime=Iload_sampletime
  Iload_6ndharmonic2 : Sin  Amplitude=Iload_peak(6)  Frequency=2*pi*Iload_freq(6)  Phase=Iload_dephase(6) + 4*pi/3*Iload_simetric(6)  SampleTime=Iload_sampletime
  Iload_6ndharmonic3 : Sin  Amplitude=Iload_peak(6)  Frequency=2*pi*Iload_freq(6)  Phase=Iload_dephase(6) + 2*pi/3*Iload_simetric(6)  SampleTime=Iload_sampletime
  Iload_6ndharmonic4 : Sin  Amplitude=Iload_peak(6)  Frequency=2*pi*Iload_freq(6)  Phase=Iload_dephase(6) + 4*pi/3*Iload_simetric(6)  SampleTime=Iload_sampletime
  Iload_6ndharmonic5 : Sin  Amplitude=Iload_peak(6)  Frequency=2*pi*Iload_freq(6)  Phase=Iload_dephase(6)  SampleTime=Iload_sampletime
  Iload_7ndharmonic : Sin  Amplitude=Iload_peak(7)  Frequency=2*pi*Iload_freq(7)  Phase=Iload_dephase(7)  SampleTime=Iload_sampletime
  Iload_7ndharmonic1 : Sin  Amplitude=Iload_peak(7)  Frequency=2*pi*Iload_freq(7)  Phase=Iload_dephase(7) + 2*pi/3*Iload_simetric(7)  SampleTime=Iload_sampletime
  Iload_7ndharmonic2 : Sin  Amplitude=Iload_peak(7)  Frequency=2*pi*Iload_freq(7)  Phase=Iload_dephase(7) + 4*pi/3*Iload_simetric(7)  SampleTime=Iload_sampletime
  Iload_7ndharmonic3 : Sin  Amplitude=Iload_peak(7)  Frequency=2*pi*Iload_freq(7)  Phase=Iload_dephase(7) + 2*pi/3*Iload_simetric(7)  SampleTime=Iload_sampletime
  Iload_7ndharmonic4 : Sin  Amplitude=Iload_peak(7)  Frequency=2*pi*Iload_freq(7)  Phase=Iload_dephase(7) + 4*pi/3*Iload_simetric(7)  SampleTime=Iload_sampletime
  Iload_7ndharmonic5 : Sin  Amplitude=Iload_peak(7)  Frequency=2*pi*Iload_freq(7)  Phase=Iload_dephase(7)  SampleTime=Iload_sampletime
  Mux5 : Mux  Inputs=3
  Scope{1..8} (8 alike) : Scope
  Sum1 : Sum  Inputs=+++++++
  Sum{3..5,7..11} (8 alike) : Sum  Inputs=+++
  Sum2 : Sum  Inputs=+++++++
  Sum6 : Sum  Inputs=+++++++
  powergui : powerlib/powergui  Priority=1  SimulationMode=Discrete  SolverType=Tustin  SampleTime=500e-9  frequency=60  SPID=off  DisableSnubberDevices=off  DisableRonSwitches=off  DisableVfSwitches=off  SwTol=0  DisplayEquations=off  Interpol=off  ExternalGateDelay=off  methode=off  Ts=10  FunctionMessages=off  echomessages=off  HookPort=off  EnableUseOfTLC=off  x0status=blocks  frequencyindice=0  Pbase=100e6  ErrMax=1e-4  Iterations=50  UnitsV=kV  UnitsW=MW  buscounter=0  RestoreLinks=warning  ResistiveCurrentMeasurement=off  Frange=[0:2:500]  Ylog=off  Xlog=on  ShowGrid=off  save=off  variable=ZData  structure=ScopeData_compensator_Subsystem__Scope10  ZoomFFT=off  StartTime=0.14  cycles=2  DisplayStyle=3  fundamental=50  FreqAxis=on  MaxFrequency=1e3  frequencyindicesteady=1  RmsSteady=1  display=off
  Out1 : Outport
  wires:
  Mux5/1 -> Out1/1
  Iload2/1 -> Sum2/1
  Iload_2ndharmonic2/1 -> Sum2/2
  Iload_6ndharmonic2/1 -> Sum2/6
  Iload_4ndharmonic2/1 -> Sum2/4
  Iload_7ndharmonic2/1 -> Sum2/7
  Iload_5ndharmonic2/1 -> Sum2/5
  Iload_3ndharmonic2/1 -> Sum2/3
  Iload1/1 -> Sum1/1
  Iload_2ndharmonic1/1 -> Sum1/2
  Iload_6ndharmonic1/1 -> Sum1/6
  Iload_5ndharmonic1/1 -> Sum1/5
  Iload_3ndharmonic1/1 -> Sum1/3
  Iload_7ndharmonic1/1 -> Sum1/7
  Iload_4ndharmonic1/1 -> Sum1/4
  Iload/1 -> Sum6/1
  Iload_2ndharmonic/1 -> Sum6/2
  Iload_5ndharmonic/1 -> Sum6/5
  Iload_7ndharmonic/1 -> Sum6/7
  Iload_3ndharmonic/1 -> Sum6/3
  Iload_6ndharmonic/1 -> Sum6/6
  Iload_4ndharmonic/1 -> Sum6/4
  Sum6/1 -> Mux5/1, Sum3/1
  Sum1/1 -> Mux5/2, Sum3/2
  Sum2/1 -> Sum3/3, Mux5/3
  Sum3/1 -> Scope1/1
  Sum4/1 -> Scope2/1
  Sum5/1 -> Scope3/1
  Sum7/1 -> Scope4/1
  Sum8/1 -> Scope5/1
  Sum9/1 -> Scope6/1
  Sum10/1 -> Scope7/1
  Iload4/1 -> Sum4/2
  Iload3/1 -> Sum4/1
  Iload5/1 -> Sum4/3
  Iload_2ndharmonic4/1 -> Sum5/2
  Iload_2ndharmonic3/1 -> Sum5/1
  Iload_2ndharmonic5/1 -> Sum5/3
  Iload_3ndharmonic5/1 -> Sum7/3
  Iload_3ndharmonic4/1 -> Sum7/2
  Iload_3ndharmonic3/1 -> Sum7/1
  Iload_4ndharmonic5/1 -> Sum8/3
  Iload_4ndharmonic4/1 -> Sum8/2
  Iload_4ndharmonic3/1 -> Sum8/1
  Iload_5ndharmonic5/1 -> Sum9/3
  Iload_5ndharmonic4/1 -> Sum9/2
  Iload_5ndharmonic3/1 -> Sum9/1
  Sum11/1 -> Scope8/1
  Iload_7ndharmonic3/1 -> Sum11/2
  Iload_7ndharmonic5/1 -> Sum11/1
  Iload_7ndharmonic4/1 -> Sum11/3
  Iload_6ndharmonic3/1 -> Sum10/2
  Iload_6ndharmonic5/1 -> Sum10/1
  Iload_6ndharmonic4/1 -> Sum10/3

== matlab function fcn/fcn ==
function [...
    Iu_ref, Iv_ref, Iw_ref,...
    activate_poles,...
    V_alpha, V_beta,... 
    control_current_start_counter_output, control_current_start_counter_max_output,...
    DVcc, DVcc_afterPI, PI_I_output...
    ] =...
    fcn(...
    Vcc_measured,...
    Ia_load, Ib_load, Ic_load,...
    Va, Vb, Vc,...
    loopPeriod,...
    k_P_DVcc, k_I_DVcc,...
    k_P_dqPLL, k_I_dqPLL,...
    Vcc_desired,...
    control_current_start_time,...
    X_C_LPF,...
    Vpeak_arbitrary)

% INPUT

% // to PLL
% Voltage phase-phase of net
% Va, Vb, Vc

% Condensator voltage:
% Vcc_measured


% Current of load measured:
% Ia_load, Ib_load, Ic_load


% OUTPUT

% Current desired to create in active filter
% Iu_ref
% Iv_ref
% Iw_ref

% output V_alpha, V_beta of dqPLL to check it keeps working, onces sure it does work these outputs are not needed
% V_alpha, V_beta

% updates of discretation



% // next lines uncomment in C: use decided value of Matlab variable
% persistent loopPeriod
% if isempty(loopPeriod)
%     loopPeriod = 10e-6; % 10 us
% end


% /* -------------------------------------------------------------------------------------- */
% // PLL

% // Tustin discretion time
persistent T_dqPLL
if isempty(T_dqPLL)
    T_dqPLL = loopPeriod;
end

% // half of Tustin discretion time. PI control Tustin use T/2, not T
persistent T_dqPLL_half
if isempty(T_dqPLL_half)
    T_dqPLL_half = T_dqPLL * 0.5;
end

% // PI control of dqPLL. Proportional constant
% persistent k_P_dqPLL
% if isempty(k_P_dqPLL)
%     k_P_dqPLL = 0.05/pi;
% end

% // PI control of dqPLL. Integral constant
% persistent k_I_dqPLL
% if isempty(k_I_dqPLL)
%     k_I_dqPLL = 0.05/pi;
% end

persistent k_I_dqPLL_Tustin
if isempty(k_I_dqPLL_Tustin)
    k_I_dqPLL_Tustin = k_I_dqPLL * T_dqPLL * 0.5; % discretion metod Tustin
end

persistent k_I_dqPLL_BE
if isempty(k_I_dqPLL_BE)
    k_I_dqPLL_BE = k_I_dqPLL * T_dqPLL; % discretion metod Backward Euler (BE)
end

% // natural frequency (rad/s) of reference of PLL (314 rad/s = 50 Hz)
persistent w_ref
if isempty(w_ref)
    w_ref = 314/pi;
end

% // Voltage q (of dq transformation) of last iteration. Needed in Tustin discretion of PI formula
persistent Vq_last
if isempty(Vq_last)
    Vq_last = 0.0;
end

% // theta used in UVW to alpha-beta transformation. At first theta is zero
persistent theta
if isempty(theta)
    theta  = 0.0;
end

% // theta used in UVW to alpha-beta transformation. At first theta is zero
% // Needed in Tustin discretion of integration of theta formula
persistent w_last
if isempty(w_last)
    w_last  = 0.0;
end

% // Tustin discretion of PI. Integral part may be saurated
persistent PI_I_dqPLL
if isempty(PI_I_dqPLL)
    PI_I_dqPLL  = 0.0;
end

% // myCos = cos(theta_rad);
% // mySin = sin(theta_rad);
% // Thus, calculate:
% // Vd = myCos * V_alpha + mySin * V_beta;
% // Vq = myCos * V_beta  - mySin * V_alpha;
% // and calculate with same values:
% // V_alpha = Vd_mean_new * myCos;
% // V_beta  = Vd_mean_new * mySin;
persistent myCos
if isempty(myCos)
    myCos  = 10.0;
end
persistent mySin
if isempty(mySin)
    mySin  = 10.0;
end

% /* -------------------------------------------------------------------------------------- */
% // discharge condensator controller

persistent T_DVcc
if isempty(T_DVcc)
    T_DVcc = loopPeriod;
end

% // next lines uncomment in C: use decided value of Matlab variable
% // dqPLL data is enough good
% persistent control_current_start
% if isempty(control_current_start)
%     control_current_start  = ...;
% end

persistent control_current_start_counter_max
if isempty(control_current_start_counter_max)
    control_current_start_counter_max = control_current_start_time/loopPeriod;
end

persistent control_current_start_counter
if isempty(control_current_start_counter)
    control_current_start_counter = 0;
end

% // next lines uncomment in C: use decided value of Matlab variable
% persistent k_P_DVcc
% if isempty(k_P_DVcc)
%     k_P_DVcc = 1e-4;
% end

% // next lines uncomment in C: use decided value of Matlab variable
% persistent k_I_DVcc
% if isempty(k_I_DVcc)
%     k_I_DVcc = 1e-3;
% end

persistent k_I_DVcc_Tustin
if isempty(k_I_DVcc_Tustin)
    k_I_DVcc_Tustin = k_I_DVcc * T_DVcc * 0.5; % discretion metod Tustin
end

% persistent Vcc_desired
% if isempty(Vcc_desired)
%     Vcc_desired = 900;
% end

persistent PI_I
if isempty(PI_I)
    PI_I = 0;
end


persistent DVcc_last
if isempty(DVcc_last)
    DVcc_last = 0;
end

persistent Gq
if isempty(Gq)
    Gq = -X_C_LPF;
end


% /* -------------------------------------------------------------------------------------- */
% // PLL


% complex_to_phase
% Vr=(Vrs-Vtr)/3;
% Vs=(Vst-Vrs)/3;
% Vt=(Vtr-Vst)/3;
Vr = (Va-Vc)/3;
Vs = (Vb-Va)/3;
Vt = (Vc-Vb)/3;
Va = Vr;
Vb = Vs;
Vc = Vt;


% matriz P1: [xalpha xbeta]'=P1*[x1 x2 x3]'
P1=[2/3 -1/3 -1/3; 0 sqrt(3)/3 -sqrt(3)/3];

V_alpha = (P1(1,:) * [Va Vb Vc]')';
V_beta  = (P1(2,:) * [Va Vb Vc]')';

% como Matlab trabaja con ángulos en rads, ej. sin(pi/2 rads) = 1, en este
% código los pablets han de convertirse en rads, pasar de [-1,1] pablets a [-pi, pi] rads
theta_rad = theta * pi;

mySin = sin(theta_rad);
myCos = cos(theta_rad);

Vd = myCos * V_alpha + mySin * V_beta;
Vq = myCos * V_beta  - mySin * V_alpha;


% /* PI controller Tustin discretion and add reference value */
% /* PI pararell   */
PI_I_dqPLL =  k_I_dqPLL_Tustin * Vq + PI_I_dqPLL;
PI_I_dqPLL =  k_I_dqPLL_Tustin * Vq_last + PI_I_dqPLL;
w = PI_I_dqPLL + k_P_dqPLL * Vq;
%             sat = 3;
%             if PI_I > sat
%                 PI_I = sat;
%             elseif PI_I < -sat
%                 PI_I = -sat;
%             end
sat = 3/pi;
if w > sat
    w = sat;
elseif w < -sat
    w = -sat;
end

w = w_ref + w;

% /* integrator Tustin discretion */
theta = T_dqPLL_half * w_last + theta;
theta = T_dqPLL_half * w + theta;

% /* update */
Vq_last = Vq;
w_last = w;

% /* output */
V_alpha = Vpeak_arbitrary * myCos;
V_beta  = Vpeak_arbitrary * mySin;
% V_alpha = Vd_dqPLL * myCos;
% V_beta  = Vd_dqPLL * mySin;


% /* -------------------------------------------------------------------------------------- */
% // discharge condensator controller

% matriz P1: [xalpha xbeta]'=P1*[x1 x2 x3]'
P1=[2/3 -1/3 -1/3; 0 sqrt(3)/3 -sqrt(3)/3];

% all current that load demands
Ialpha_load = (P1(1,:) * [Ia_load, Ib_load, Ic_load]')';
Ibeta_load  = (P1(2,:) * [Ia_load, Ib_load, Ic_load]')';


if control_current_start_counter > control_current_start_counter_max
    DVcc = Vcc_desired - Vcc_measured;
    activate_poles = 1;
else
    control_current_start_counter = 1 + control_current_start_counter;
    DVcc = 0;
    activate_poles = 0;
end

% /* PI controller Tustin discretion */
% /* PI pararell   */
PI_I =  k_I_DVcc_Tustin * DVcc + PI_I;
PI_I =  k_I_DVcc_Tustin * DVcc_last + PI_I;
DVcc_afterPI = PI_I + k_P_DVcc * DVcc;
%             sat = 3;
%             if PI_I > sat
%                 PI_I = sat;
%             elseif PI_I < -sat
%                 PI_I = -sat;
%             end
sat = 1e3;
if DVcc_afterPI > sat
    DVcc_afterPI = sat;
elseif DVcc_afterPI < -sat
    DVcc_afterPI = -sat;
end

% discharge of condensators which power the active filter
I_compensate_ref_phase_alpha_because_DVcc = Ialpha_load - V_alpha * DVcc_afterPI ;
I_compensate_ref_phase_beta_because_DVcc  = Ibeta_load  - V_beta  * DVcc_afterPI ;

% Reactive of condensator of LPF of active filter
I_alpha_desired_compensate_PQ =  Gq * V_beta;
I_beta_desired_compensate_PQ  = -Gq * V_alpha;
% I_alpha_desired_compensate_PQ = 0;
% I_beta_desired_compensate_PQ = 0;

% sum of currents to compensate
Ialpha_ref = I_compensate_ref_phase_alpha_because_DVcc + I_alpha_desired_compensate_PQ ;
Ibeta_ref  = I_compensate_ref_phase_beta_because_DVcc  + I_beta_desired_compensate_PQ  ;


% /* update */
DVcc_last = DVcc;


% /* output */
% AlphaBeta to abc
Iu_ref = Ialpha_ref;
Iv_ref = -.5 * Ialpha_ref + .866 * Ibeta_ref;
Iw_ref = -.5 * Ialpha_ref - .866 * Ibeta_ref;

% to check
control_current_start_counter_output = control_current_start_counter;
control_current_start_counter_max_output = control_current_start_counter_max;
PI_I_output = PI_I;

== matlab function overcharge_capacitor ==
function pSfrenado  = overcharge_capacitor(Vcc_measured, Vcc_upperlimit, Vcc_lowerlimit)

persistent pS;
if ( isempty(pS) )
    pS = 0;
end


% Sliding on currents
if (Vcc_measured > Vcc_upperlimit)
    pS = 1;
elseif (Vcc_measured < Vcc_lowerlimit)
    pS = 0;
% else
    % mantain value cause it is 'persistent'
end

% output in Matlab cannot be a persistent
pSfrenado = pS;
return

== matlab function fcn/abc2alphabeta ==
function [alpha, beta] = abc_AlphaBetaGamma(a, b, c)

k1 = 2 / 3;
k2 = 1 / 3;
k3 = sqrt(3) / 3;

alpha = a * k1 - b * k2 - c * k2;
beta  =          b * k3 - c * k3;
% gamma = a * k2 + b * k2 + c * k2;
    
%end function

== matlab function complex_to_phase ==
function [Vr,Vs,Vt] = complex_to_phase(Vrs,Vst,Vtr)

if ( isempty(Vrs) || isempty(Vst) || isempty(Vtr) )
    Vrs = 0;
    Vst = 0;
    Vtr = 0;
end

Vr=(Vrs-Vtr)/3;
Vs=(Vst-Vrs)/3;
Vt=(Vtr-Vst)/3;

% % Vrs=Vr-Vs
% % Vst=Vs-Vt
% % Vtr=Vt-Vr
% % Así que A*y=x=[Vr,Vs,Vt]'
% % A=[ 1 -1 0;...
% %     0 1 -1;...
% %     -1 0 1];
% % B=[Vrs Vst Vtr]';
% % NO TVENE SOLUCVÓN
% 
% 
% % Suponemos que hubVera neutro: Vr+Vs+Vt=0
% A=[ 1 -1 0;...
%     0 1 -1;...
%     1 1 1];
% B=[Vrs Vst 0]';
% 
% X=lVnsolve(A,B);% solves the linear system A*X=B
% 
% Vr=X(1);
% Vs=X(2);
% Vt=X(3);

return

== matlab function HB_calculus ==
function HB  = HB_calculus(Vfaseneutro , Kh, Vcc_desired)

Vrn = Vfaseneutro(1);
Vsn = Vfaseneutro(2);
Vtn = Vfaseneutro(3);

HB = zeros(3,1);
HB(1) = Kh * ( (Vcc_desired/2)^2 - Vrn^2 );
HB(2) = Kh * ( (Vcc_desired/2)^2 - Vsn^2 );
HB(3) = Kh * ( (Vcc_desired/2)^2 - Vtn^2 );

return

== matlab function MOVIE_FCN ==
function [a1,b1,c1,d1,e1,f1,g1]  = MOVIE_FCN(a,b,c,d,e,f,g)

a1 = a;
b1 = b;
c1 = c;
d1 = d;
e1 = e;
f1 = f;
g1 = g;


return

== matlab function measured&desired_to_SuSvSw/Embedded
MATLAB Function ==
function [Su, Sv, Sw] = sliding(Iu, Iv, Iw, Iu1, Iv1, Iw1, H)

if ( isempty(Iu) )%|| isempty(Iv) || isempty(Iw) )
    Iu = 0;
    Iv = 0;
    Iw = 0;
end

persistent pSu pSv pSw;
if ( isempty(pSu) )%|| isempty(pSv) || isempty(pSw) )
    pSu = 0;
    pSv = 0;
    pSw = 0;
end

Hu = H(1);
Hv = H(2);
Hw = H(3);

% Sliding on currents
if (Iu >= (Iu1+Hu))
    pSu = 0;
elseif (Iu < (Iu1-Hu))
    pSu = 1;
% else (Iu1 < (Iu+H)) & (Iu1 >= (Iu-H))
    % pSu mantain value cause it is 'persistent'
end

if (Iv >= (Iv1+Hv))
    pSv = 0;
elseif (Iv < (Iv1-Hv))
    pSv = 1;
end

if (Iw >= (Iw1+Hw))
    pSw = 0;
elseif (Iw < (Iw1-Hw))
    pSw = 1;
end

% Inverter state
Su = pSu;
Sv = pSv;
Sw = pSw;

% comprobar q disparo es On ó Off
% if ~(Su==0 || Su==1) % if it is NOT 0 or 1
%     error('error Su is not right')
% end
% if ~(Sv==0 || Sv==1) 
%     error('error Sv is not right')
% end
% if ~(Sw==0 || Sw==1) 
%     error('error Sw is not right')
% end

return

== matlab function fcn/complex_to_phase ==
function [Vr,Vs,Vt] = complex_to_phase(Vrs,Vst,Vtr)

if ( isempty(Vrs) || isempty(Vst) || isempty(Vtr) )
    Vrs = 0;
    Vst = 0;
    Vtr = 0;
end

Vr=(Vrs-Vtr)/3;
Vs=(Vst-Vrs)/3;
Vt=(Vtr-Vst)/3;

% % Vrs=Vr-Vs
% % Vst=Vs-Vt
% % Vtr=Vt-Vr
% % Así que A*y=x=[Vr,Vs,Vt]'
% % A=[ 1 -1 0;...
% %     0 1 -1;...
% %     -1 0 1];
% % B=[Vrs Vst Vtr]';
% % NO TVENE SOLUCVÓN
% 
% 
% % Suponemos que hubVera neutro: Vr+Vs+Vt=0
% A=[ 1 -1 0;...
%     0 1 -1;...
%     1 1 1];
% B=[Vrs Vst 0]';
% 
% X=lVnsolve(A,B);% solves the linear system A*X=B
% 
% Vr=X(1);
% Vs=X(2);
% Vt=X(3);

return
